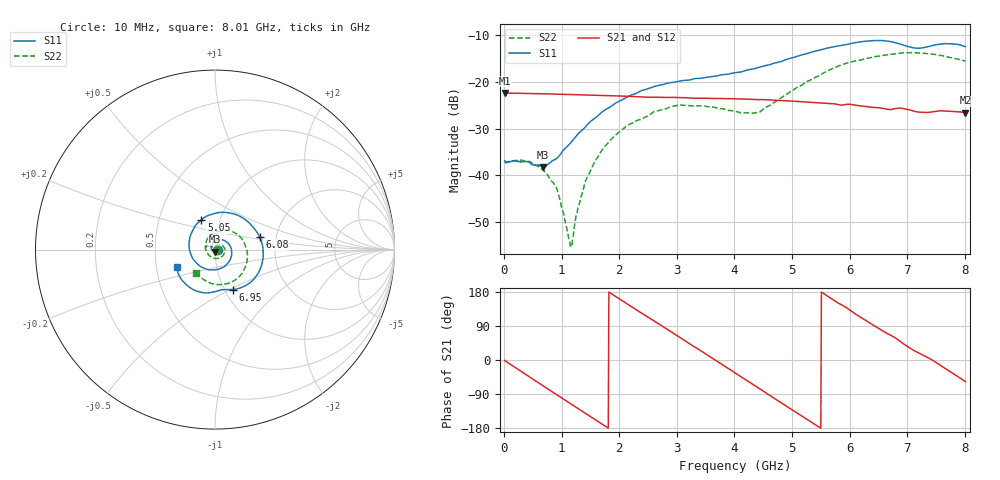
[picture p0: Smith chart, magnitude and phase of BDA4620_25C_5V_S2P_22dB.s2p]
!Agilent Technologies,E5071B,MY42404982,A.09.10
!Date: Wed May 06 09:03:06 2026
!Data & Calibration Information:
!Freq	S11:SOLT2(ON)	S21:SOLT2(ON)	S12:SOLT2(ON)	S22:SOLT2(ON)
# Hz S RI R 50
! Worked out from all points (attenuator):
!   801 points, 10 MHz to 8.01 GHz, reference 50 ohm
!   highest |S21| = -22.40 dB at 10 MHz (marker M1); lowest = -26.6 dB at 8.01 GHz (marker M2)
!   lowest |S11| = -38.2 dB at 680 MHz (marker M3), VSWR 1.02, Z = 49.7 - j1.19 ohm
!   |S11| at or under -10 dB: start of sweep to end of sweep
!   |S22| runs from -55.1 to -13.8 dB; largest |S21 - S12| = 0.00041
!   S11 on the Smith chart (normalised r, x): 10 MHz: 1.03, -0.00; 5.05 GHz: 0.82, +0.28; 6.08 GHz: 1.64, +0.25; 6.95 GHz: 1.09, -0.52; 8.01 GHz: 0.64, -0.13
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1e7  0.0143 -0.000959  0.0758 -0.00162  0.0759 -0.00165  0.0136 -0.000479
4.2e8  0.00819 -0.0113  0.0552 -0.0503  0.0553 -0.0505  0.0133 -0.00476
6.8e8  -0.00247 -0.012  0.0275 -0.0688  0.0275 -0.069  0.00911 -0.00674
9.2e8  -0.0139 -0.00629  -0.00267 -0.0734  -0.00274 -0.0735  0.00358 -0.00609
1.15e9  -0.0209 0.00683  -0.0307 -0.0661  -0.0308 -0.0662  -0.00137 -0.00114
1.19e9  -0.0214 0.00974  -0.0351 -0.0637  -0.0352 -0.0638  -0.00206 0.000118
1.26e9  -0.0219 0.0149  -0.0423 -0.0588  -0.0425 -0.0589  -0.00314 0.00227
1.35e9  -0.0212 0.0216  -0.0507 -0.0514  -0.0509 -0.0514  -0.00365 0.00503
1.54e9  -0.0148 0.0363  -0.064 -0.0322  -0.0641 -0.0322  -0.0033 0.0122
1.77e9  0.00165 0.0505  -0.0708 -0.00515  -0.0709 -0.00512  0.000941 0.021
2.15e9  0.043 0.0541  -0.0584 0.0381  -0.0585 0.0382  0.0176 0.0296
2.68e9  0.0909 0.00464  -0.0068 0.0677  -0.00675 0.0678  0.0451 0.0191
3.07e9  0.0837 -0.0581  0.036 0.0572  0.0361 0.0572  0.0559 -0.00714
4.01e9  -0.0845 -0.0912  0.0544 -0.0366  0.0545 -0.0368  -0.0114 -0.047
4.42e9  -0.1418 -0.00294  0.0177 -0.0618  0.0176 -0.0619  -0.0458 -0.0127
5.05e9  -0.076 0.1659  -0.0445 -0.0428  -0.0447 -0.0428  -0.0256 0.0798
5.35e9  0.0192 0.2063  -0.0581 -0.0151  -0.0581 -0.0151  0.0234 0.1032
6.08e9  0.2485 0.0711  -0.0312 0.047  -0.0311 0.0471  0.1586 0.0459
6.68e9  0.1976 -0.1826  0.0191 0.0467  0.0192 0.0468  0.1709 -0.0912
6.95e9  0.098 -0.2224  0.0386 0.0339  0.0388 0.0338  0.1354 -0.1504
7.58e9  -0.0878 -0.2353  0.0472 -0.0122  0.0474 -0.012  -0.0188 -0.1888
8.01e9  -0.2134 -0.0995  0.0254 -0.039  0.0255 -0.039  -0.1046 -0.128
